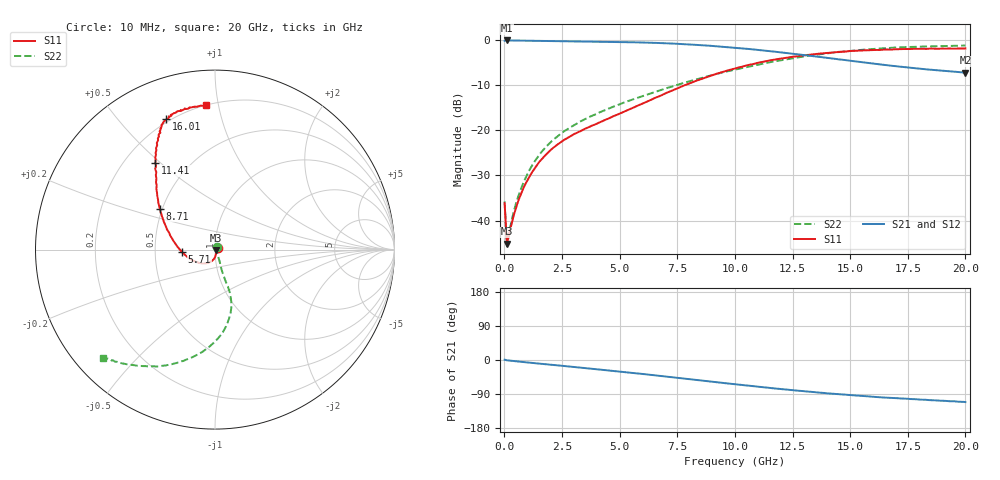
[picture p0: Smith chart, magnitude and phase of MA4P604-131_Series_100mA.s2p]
! AWR Design Environment (9226) Thu Aug 19 15:08:55 2021
! Document = '100mA'
! nPorts: 2, nXvals: 201
# GHz S DB R 50
!Freq DBS11 AngS11 DBS21 AngS21 DBS12 AngS12 DBS22 AngS22
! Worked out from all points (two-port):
!   201 points, 10 MHz to 20 GHz, reference 50 ohm
!   highest |S21| = -0.10 dB at 110 MHz (marker M1); lowest = -7.2 dB at 20 GHz (marker M2)
!   |S21| within 3 dB of the highest: start of sweep to 12.61 GHz
!   lowest |S11| = -45.1 dB at 110 MHz (marker M3), VSWR 1.01, Z = 50.5 - j0.192 ohm
!   |S11| at or under -10 dB: start of sweep to 7.83 GHz
!   |S22| runs from -45.7 to -1.2 dB; largest |S21 - S12| = 0.028
!   S11 on the Smith chart (normalised r, x): 10 MHz: 1.03, +0.01; 5.71 GHz: 0.69, -0.02; 8.71 GHz: 0.48, +0.26; 11.41 GHz: 0.33, +0.48; 16.01 GHz: 0.19, +0.68; 20 GHz: 0.20, +0.92
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0.01  -36.13 24.2  -0.18 0.8  -0.13 0.8  -35.75 54.2
0.11  -45.12 -20.1  -0.10 -0.8  -0.08 -0.8  -45.67 -21.7
0.31  -40.80 -48.5  -0.11 -2.1  -0.09 -2.1  -40.04 -44.7
0.51  -37.13 -62.5  -0.12 -3.4  -0.10 -3.3  -36.08 -55.1
0.81  -33.00 -74.4  -0.14 -5.3  -0.12 -5.2  -31.81 -60.4
1.21  -29.22 -84.6  -0.17 -7.7  -0.15 -7.5  -27.74 -64.6
1.61  -26.47 -93.3  -0.20 -10.1  -0.18 -9.9  -24.81 -67.1
2.11  -23.92 -103.9  -0.23 -13.0  -0.22 -12.7  -22.15 -69.7
2.61  -22.06 -114.3  -0.26 -16.0  -0.24 -15.6  -20.15 -71.1
3.41  -19.88 -130.2  -0.31 -20.8  -0.29 -20.2  -17.77 -71.8
4.71  -16.93 -156.4  -0.41 -28.6  -0.40 -28.0  -14.80 -71.5
5.71  -14.70 -175.6  -0.52 -35.0  -0.50 -34.2  -12.90 -70.8
6.71  -12.47 167.7  -0.66 -41.6  -0.65 -40.7  -11.22 -71.6
8.71  -8.33 143.3  -1.20 -55.2  -1.17 -53.9  -8.19 -78.3
10.01  -6.31 132.2  -1.71 -64.2  -1.65 -62.5  -6.58 -85.3
11.41  -4.63 124.5  -2.40 -73.1  -2.30 -71.5  -5.03 -95.5
13.41  -3.15 117.3  -3.58 -84.5  -3.43 -83.3  -3.35 -110.3
16.01  -2.22 110.5  -5.22 -97.1  -5.13 -96.2  -1.98 -126.2
16.71  -2.13 108.5  -5.65 -99.9  -5.60 -99.0  -1.75 -129.1
18.21  -1.96 103.9  -6.45 -104.6  -6.51 -104.4  -1.44 -133.7
19.51  -1.92 97.5  -7.01 -108.9  -7.19 -108.4  -1.29 -135.4
20  -1.87 93.7  -7.24 -111.0  -7.47 -109.8  -1.23 -135.8
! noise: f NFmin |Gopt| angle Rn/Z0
0.01  0  1  0  2e-20
2.21  0  1  0  2e-20
4.41  0  1  0  2e-20
6.61  0  1  0  2e-20
8.81  0  1  0  2e-20
11.11  0  1  0  2e-20
13.31  0  1  0  2e-20
15.51  0  1  0  2e-20
17.71  0  1  0  2e-20
20  0  1  0  2e-20
